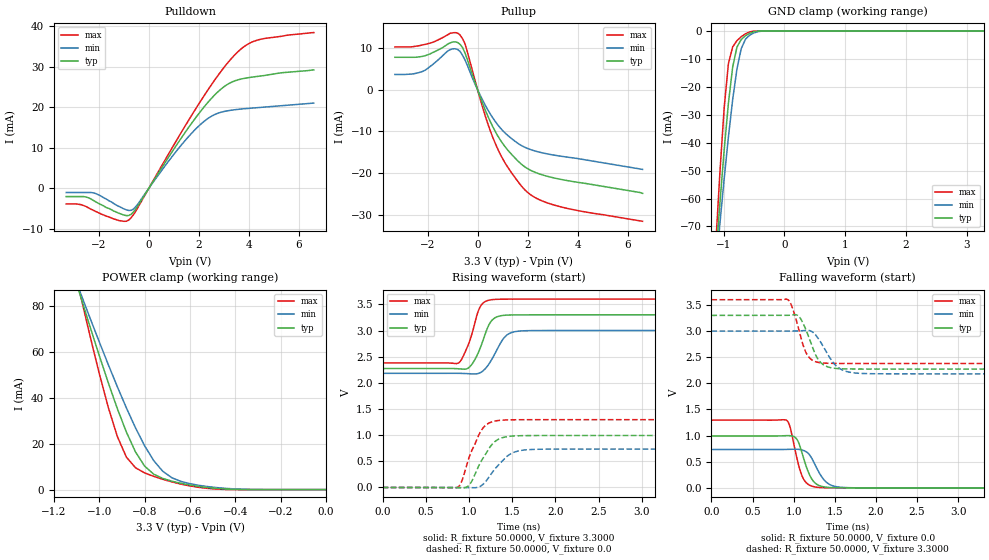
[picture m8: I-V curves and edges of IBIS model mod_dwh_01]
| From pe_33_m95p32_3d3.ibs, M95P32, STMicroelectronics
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|   Model mod_dwh_01
[Model]   mod_dwh_01
Model_type I/O
Polarity   Non-Inverting
Vinl   =   1.000V
Vinh   =   2.300V
Vmeas  =   1.650V
Cref   =   30pF
C_comp   1.607pF   1.535pF   1.683pF
[Model Spec]
Vinl   1.000V  0.900V  1.080V  | <- for Vcc = 3.3V, 3.0V, 3.6V
Vinh   2.300V  2.100V  2.520V  | <- for Vcc = 3.3V, 3.0V, 3.6V
Vmeas  1.650V  1.500V  1.800V  | <- for Vcc = 3.3V, 3.0V, 3.6V
[Temperature Range]   25.0000   0.1050k   -40.0000
[Voltage Range]   3.3000V   3.0000V   3.6000V
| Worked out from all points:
|   slope of the pulldown table from 0 to 0.495 V, typ, clamps not added: 102 ohm
|   slope of the pullup table from 0 to 0.495 V, typ, clamps not added: 66.2 ohm
|   GND clamp passes 1 mA (typ) near -0.58 V on its own axis
|   POWER clamp passes 1 mA (typ) near -0.53 V on its own axis
|   rising waveform, R_fixture 50.0000, V_fixture 3.3000: 20-80 % time 148ps typ, 170ps min, 139ps max; typ from 2.27 V to 3.3 V
|   rising waveform, R_fixture 50.0000, V_fixture 0.0: 20-80 % time 197ps typ, 224ps min, 180ps max; typ from 0 V to 0.993 V
|   falling waveform, R_fixture 50.0000, V_fixture 0.0: 20-80 % time 133ps typ, 161ps min, 119ps max; typ from 0.993 V to 0 V
|   falling waveform, R_fixture 50.0000, V_fixture 3.3000: 20-80 % time 159ps typ, 201ps min, 136ps max; typ from 3.3 V to 2.27 V
[Pulldown]
|Voltage   I(typ)   I(min)   I(max)
-3.3V     -2mA       -1mA       -3.8mA
-2.7V     -2mA       -1mA       -4mA
-2.2V     -3mA       -1.1mA     -5.41mA
-1.2V     -6.1mA     -4.4mA     -7.9mA
-800mV    -6.672mA   -5.427mA   -7.788mA
-500mV    -4.897mA   -4.364mA   -5.402mA
1V        9.644mA    8.367mA    10.67mA
2V        18.41mA    15.37mA    20.81mA
2.8V      23.99mA    18.61mA    28.09mA
3.5V      26.63mA    19.43mA    33.27mA
4.4V      27.64mA    19.93mA    36.63mA
6.6V      29.2mA     21.03mA    38.4mA
[Pullup]
|Voltage   I(typ)   I(min)   I(max)
-3.3V     7.74mA     3.62mA     10.21mA
-2.2V     7.962mA    4.344mA    10.7mA
-1.2V     10.88mA    9.22mA     13.11mA
-800mV    11.29mA    9.63mA     13.55mA
-500mV    8.759mA    7.095mA    10.97mA
200mV     -3.257mA   -2.493mA   -4.198mA
700mV     -9.953mA   -7.585mA   -12.78mA
1.2V      -14.45mA   -10.95mA   -18.55mA
1.9V      -18.58mA   -13.87mA   -24.1mA
2.4V      -20.08mA   -14.9mA    -26.22mA
3.2V      -21.38mA   -15.86mA   -27.93mA
6.6V      -24.9mA    -19.15mA   -31.6mA
[GND_clamp]
|Voltage   I(typ)   I(min)   I(max)
-3.3V     -807.6mA   -672mA     -1.053A
-1.13V    -81.94mA   -85.75mA   -76.94mA
-1.06V    -61.58mA   -68.96mA   -50.51mA
-990mV    -42.58mA   -52.9mA    -27.53mA
-920mV    -25.81mA   -37.91mA   -11.64mA
-850mV    -12.88mA   -24.52mA   -5.709mA
-780mV    -5.82mA    -13.61mA   -3.523mA
-710mV    -3.106mA   -6.377mA   -2.091mA
-640mV    -1.742mA   -2.986mA   -1.046mA
-500mV    -309.6uA   -721.8uA   -69.16uA
-290mV    -791nA     -10.61uA   -17.06nA
3.28V     561.4pA    18.21uA    173.1pA
[POWER_clamp]
|Voltage   I(typ)   I(min)   I(max)
-3.28V    853.2mA    705.5mA    1.123A
-1.08V    83.64mA    85.1mA     83.66mA
-1V       58.53mA    64.51mA    50.75mA
-960mV    46.59mA    54.53mA    35.87mA
-920mV    35.3mA     44.85mA    23.13mA
-880mV    25.04mA    35.59mA    14.12mA
-840mV    16.42mA    26.93mA    9.512mA
-800mV    10.26mA    19.14mA    7.302mA
-720mV    4.876mA    8.001mA    4.493mA
-640mV    2.758mA    3.578mA    2.397mA
-400mV    94.29uA    284.7uA    12.64uA
0V        840.7pA    17.31nA    345.8pA
[Ramp]
| variable   typ   min   max
dV/dt_r  0.5960/0.2466n   0.4547/0.2831n   0.7775/0.2624n
dV/dt_f  0.6158/0.2584n   0.5035/0.2926n   0.7319/0.2207n
R_load = 50.0000
[Rising Waveform]
R_fixture= 50.0000
V_fixture= 3.3000
V_fixture_min= 3.0000
V_fixture_max= 3.6000
|time   V(typ)   V(min)   V(max)
0s        2.274V     2.182V     2.38V
880ps     2.269V     2.182V     2.38V
928ps     2.262V     2.18V      2.493V
1.008ns   2.306V     2.173V     2.801V
1.12ns    2.626V     2.186V     3.424V
1.216ns   3.058V     2.326V     3.574V
1.264ns   3.193V     2.45V      3.59V
1.424ns   3.293V     2.893V     3.599V
1.6ns     3.299V     2.992V     3.6V
6ns       3.3V       3V         3.6V
[Rising Waveform]
R_fixture= 50.0000
V_fixture= 0.0
V_fixture_min= 0.0
V_fixture_max= 0.0
|time   V(typ)   V(min)   V(max)
0s        10.02nV    1.042uV    1.807nV
872ps     -1.967mV   349.7uV    5.457mV
920ps     -5.369mV   -148.6uV   137.8mV
1ns       42.52mV    -2.564mV   574.8mV
1.144ns   512.4mV    35.72mV    1.096V
1.256ns   802.4mV    257.4mV    1.25V
1.336ns   917.6mV    421.5mV    1.28V
1.496ns   981.9mV    655.8mV    1.294V
1.736ns   992.6mV    727.5mV    1.296V
6ns       993.3mV    733.9mV    1.296V
[Falling Waveform]
R_fixture= 50.0000
V_fixture= 0.0
V_fixture_min= 0.0
V_fixture_max= 0.0
|time   V(typ)   V(min)   V(max)
0s        993.3mV    733.9mV    1.296V
912ps     999.2mV    735.7mV    1.296V
960ps     997.6mV    737.8mV    1.144V
1.04ns    929.5mV    738.6mV    565.1mV
1.104ns   657.1mV    724.1mV    221.3mV
1.2ns     227.1mV    617.6mV    45.74mV
1.28ns    69.27mV    381.3mV    12.68mV
1.408ns   10.82mV    95.05mV    1.663mV
1.616ns   587.2uV    6.922mV    71.71uV
6ns       1.44uV     2.318uV    1.623uV
[Falling Waveform]
R_fixture= 50.0000
V_fixture= 3.3000
V_fixture_min= 3.0000
V_fixture_max= 3.6000
|time   V(typ)   V(min)   V(max)
0s        3.3V       3V         3.6V
936ps     3.302V     3V         3.596V
984ps     3.308V     3V         3.449V
1.048ns   3.301V     3.002V     3.119V
1.144ns   3.046V     3.013V     2.609V
1.224ns   2.71V      2.988V     2.446V
1.32ns    2.413V     2.81V      2.395V
1.528ns   2.283V     2.32V      2.381V
1.768ns   2.274V     2.195V     2.38V
6ns       2.274V     2.182V     2.38V
